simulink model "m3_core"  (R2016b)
settings: Solver=FixedStepDiscrete  StartTime=0.0  StopTime=inf  RelTol=1e-3  EnableMultiTasking=on
libraries: f28M36x_M3_lib x3

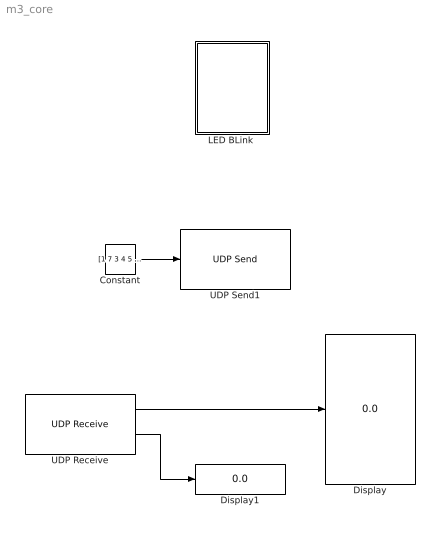
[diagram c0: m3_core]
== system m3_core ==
  Constant : Constant  Value=[1 7 3 4 5 7 7 8]  OutDataTypeStr=uint16
  Display : Display
  Display1 : Display
  "LED BLink " : Subsystem
  UDP Receive : f28M36x_M3_lib/UDP Receive  LocalIPPort_=25555  RemoteIPAddress_=0.0.0.0  DataType=uint16  DataLength=8  BlockingMode=off  SampleTime=0.1
  UDP Send1 : f28M36x_M3_lib/UDP Send  RemoteIPAddress_=255.255.255.255  RemoteIPPort_=25000  LocalIPPort_=-1  BlockingMode=off
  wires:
  Constant/1 -> UDP Send1/1
  UDP Receive/1 -> Display/1
  UDP Receive/2 -> Display1/1

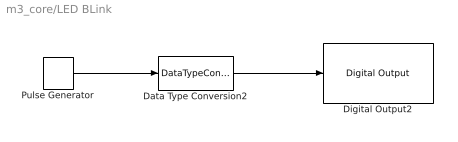
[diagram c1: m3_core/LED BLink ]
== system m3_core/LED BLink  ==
  Data Type Conversion2 : DataTypeConversion  OutDataTypeStr=boolean
  Digital Output2 : f28M36x_M3_lib/Digital Output  gpio_name=GPIOC  pin_number=7  pupd_reg=0  otype_reg=0  ospeed_reg=0  gpio_init_out=on  toggle_pin=on
  Pulse Generator : DiscretePulseGenerator  PulseType=Time based  Period=0.5  PulseWidth=50
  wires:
  Data Type Conversion2/1 -> Digital Output2/1
  Pulse Generator/1 -> Data Type Conversion2/1
